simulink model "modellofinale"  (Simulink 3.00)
settings: Solver=ode45  StartTime=0.0  StopTime=10.0  RelTol=1e-3
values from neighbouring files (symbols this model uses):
  a = u(9)    [acceler.m]    (also in Dati2lin.m = 1; cin_inversa.m = u(4))
  b1 = 1    [Dati2lin.m]
  b2 = 1    [Dati2lin.m]
  Del1 = 0.0022    [Dati2lin.m]
  Del2 = 0.0022    [Dati2lin.m]
  Dm1 = 0.000172    [Dati2lin.m]
  Dm2 = 0.000071    (= 7.1e-05)    [Dati2lin.m]
  g = u(10)    [acceler.m]    (also in Dati2lin.m = 9.806)
  Jm1 = 0.000656    [Dati2lin.m]
  Jm2 = 0.000027    (= 2.7e-05)    [Dati2lin.m]
  Kcp1 = 32    [Dati2lin.m]
  Kcp2 = 32    [Dati2lin.m]
  Kcv1 = 0.24275    [Dati2lin.m]
  Kcv2 = 0.029363    [Dati2lin.m]
  Kel1 = 36.3    [Dati2lin.m]
  Kel2 = 4.6    [Dati2lin.m]
  Kt1 = 1.75    [Dati2lin.m]
  Kt2 = 0.97    [Dati2lin.m]
  m1 = u(7)    [acceler.m]    (also in Dati2lin.m = 19)
  m2 = u(8)    [acceler.m]    (also in Dati2lin.m = 9)
  n1 = 100    [Dati2lin.m]
  n2 = 100    [Dati2lin.m]
  q01 = atan2(s1,c1)    [traiettoria1.m]    (also in traiettoria2.m; traiettoria3.m; Dati2lin.m = 0)
  q02 = atan2(s2,c2)    [traiettoria1.m]    (also in traiettoria2.m; traiettoria3.m; Dati2lin.m = 0)
  qm01 = n1*q01 + taulm01/Kel1    [traiettoria1.m]    (also in traiettoria2.m; traiettoria3.m; Dati2lin.m)
  qm02 = n2*q02 + taulm02/Kel2    [traiettoria1.m]    (also in traiettoria2.m; traiettoria3.m; Dati2lin.m)
  Tiv1 = 25    [Dati2lin.m]
  Tiv2 = 5.2632    [Dati2lin.m]
  u01 = taulm01/Kt1    [traiettoria1.m]    (also in traiettoria2.m; traiettoria3.m; Dati2lin.m)
  u02 = taulm02/Kt2    [traiettoria1.m]    (also in traiettoria2.m; traiettoria3.m; Dati2lin.m)

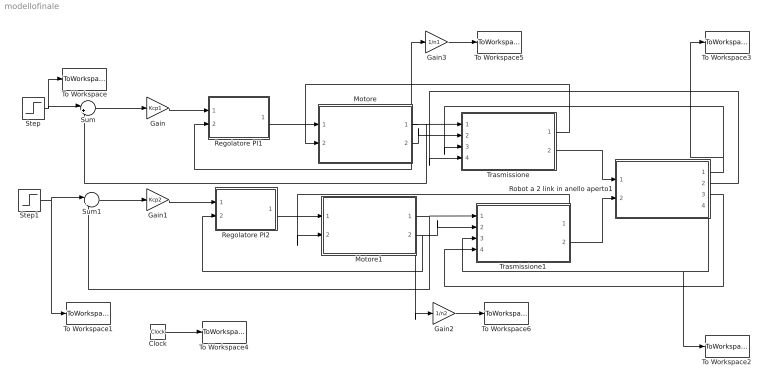
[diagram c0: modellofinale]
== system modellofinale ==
  Clock : Clock
  Gain : Gain  Gain=Kcp1  SaturateOnIntegerOverflow=on
  Gain1 : Gain  Gain=Kcp2  SaturateOnIntegerOverflow=on
  Gain2 : Gain  Gain=1/n2  SaturateOnIntegerOverflow=on
  Gain3 : Gain  Gain=1/n1  SaturateOnIntegerOverflow=on
  Motore : Subsystem  mask(Motore (solo meccanica)){Kt=Kt1, Jm=Jm1, Dm=Dm1, Qm0=qm01}
      mask prompts: Kt "Costante di coppia (Kt)"; Jm "Momento d'inerzia (Jm)"; Dm "Coefficiente di attrito viscoso (Dm)"; Qm0 "Posizione iniziale (Qm0)"
      mask help: Motore controllato in tensione - Modello che tiene conto degli effetti dell'attrito (solo quello viscoso)
  Motore1 : Subsystem  mask(Motore (solo meccanica)){Kt=Kt2, Jm=Jm2, Dm=Dm2, Qm0=qm02}
      mask prompts: Kt "Costante di coppia (Kt)"; Jm "Momento d'inerzia (Jm)"; Dm "Coefficiente di attrito viscoso (Dm)"; Qm0 "Posizione iniziale (Qm0)"
      mask help: Motore controllato in tensione - Modello che tiene conto degli effetti dell'attrito (solo quello viscoso)
  Regolatore PI1 : Subsystem  mask(Controllore PID ISA){Kc=Kcv1, Ti=Tiv1, b=b1, p6=[-inf,inf], u0=u01}
      mask prompts: Kc "Guadagno (Kc)"; Ti "Tempo integrale (Ti)"; b "Peso sul setpoint (b)"; p6 "Saturazione antiwindup ([umin, umax])"; u0 "Variabile di controllo iniziale (u0)"
      mask init:
      | ulow = p6(1);
      | uhigh = p6(2);
  Regolatore PI2 : Subsystem  mask(Controllore PID ISA){Kc=Kcv2, Ti=Tiv2, b=b2, p6=[-inf,inf], u0=u02}
      mask prompts: Kc "Guadagno (Kc)"; Ti "Tempo integrale (Ti)"; b "Peso sul setpoint (b)"; p6 "Saturazione antiwindup ([umin, umax])"; u0 "Variabile di controllo iniziale (u0)"
      mask init:
      | ulow = p6(1);
      | uhigh = p6(2);
  Robot a 2 link in anello aperto1 : Subsystem  mask(Modello del robot planare a 2 link){m1=m1, m2=m2, a=a, q01=q01, q02=q02, g=g}
      mask prompts: m1 "Massa del link 1 (m1)"; m2 "Massa del link 2 (m2)"; a "Lunghezza del link (a)"; q01 "Posizione iniziale link 1 (q01)"; q02 "Posizione iniziale link 2 (q02)"; g "Accelerazione di gravità (g)"
  Step : Step  Time=0  Before=0  After=0  SampleTime=0
  Step1 : Step  Time=0.1  Before=0  After=n2  SampleTime=0
  Sum : Sum  Inputs=|+-  SaturateOnIntegerOverflow=on
  Sum1 : Sum  Inputs=|+-  SaturateOnIntegerOverflow=on
  To Workspace : ToWorkspace  VariableName=step1  SampleTime=-1  SaveFormat=Matrix
  To Workspace1 : ToWorkspace  VariableName=step2  SampleTime=-1  SaveFormat=Matrix
  To Workspace2 : ToWorkspace  VariableName=qout2  SampleTime=-1  SaveFormat=Matrix
  To Workspace3 : ToWorkspace  VariableName=qout1  SampleTime=-1  SaveFormat=Matrix
  To Workspace4 : ToWorkspace  VariableName=x  SampleTime=-1  SaveFormat=Matrix
  To Workspace5 : ToWorkspace  VariableName=qmout1  SampleTime=-1  SaveFormat=Matrix
  To Workspace6 : ToWorkspace  VariableName=qmout2  SampleTime=-1  SaveFormat=Matrix
  Trasmissione : Subsystem  mask(Riduttore){n=n1, Kel=Kel1, Del=Del1}
      mask prompts: n "Rapporto di trasmissione (n)"; Kel "Coefficiente di elasticità (Kel)"; Del "Coefficiente di smorzamento (Del)"
      mask help: Riduttore - Modello che tiene conto dei soli effetti elastici (senza considerare le inerzie, accorpate nel modello del motore) e di un termine di smorzamento
  Trasmissione1 : Subsystem  mask(Riduttore){n=n2, Kel=Kel2, Del=Del2}
      mask prompts: n "Rapporto di trasmissione (n)"; Kel "Coefficiente di elasticità (Kel)"; Del "Coefficiente di smorzamento (Del)"
      mask help: Riduttore - Modello che tiene conto dei soli effetti elastici (senza considerare le inerzie, accorpate nel modello del motore) e di un termine di smorzamento
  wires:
  Sum/1 -> Gain/1
  Sum1/1 -> Gain1/1
  Gain/1 -> Regolatore PI1/1(ysp)
  Gain1/1 -> Regolatore PI2/1(ysp)
  Regolatore PI1/1(u) -> Motore/1(I)
  Regolatore PI2/1(u) -> Motore1/1(I)
  Trasmissione/2("tau_ll ") -> Robot a 2 link in anello aperto1/1(taull1)
  Trasmissione1/2("tau_ll ") -> Robot a 2 link in anello aperto1/2(taull2)
  Trasmissione1/1("tau_lm ") -> Motore1/2(tau_lm)
  Robot a 2 link in anello aperto1/3(dq2) -> Trasmissione1/4("dq ")
  Robot a 2 link in anello aperto1/2(dq1) -> Trasmissione/4("dq ")
  Trasmissione/1("tau_lm ") -> Motore/2(tau_lm)
  Motore1/2(dqm) -> Trasmissione1/2(dqm), Regolatore PI2/2(y)
  Motore/2(dqm) -> Trasmissione/2(dqm), Regolatore PI1/2(y)
  Motore/1(qm) -> Trasmissione/1(qm), Sum/2, Gain3/1
  Motore1/1(qm) -> Trasmissione1/1(qm), Sum1/2, Gain2/1
  Step/1 -> Sum/1, To Workspace/1
  Step1/1 -> Sum1/1, To Workspace1/1
  Robot a 2 link in anello aperto1/1(q1) -> Trasmissione/3("q "), To Workspace3/1
  Robot a 2 link in anello aperto1/4(q2) -> Trasmissione1/3("q "), To Workspace2/1
  Clock/1 -> To Workspace4/1
  Gain3/1 -> To Workspace5/1
  Gain2/1 -> To Workspace6/1

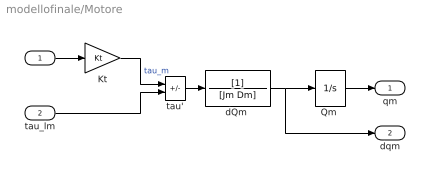
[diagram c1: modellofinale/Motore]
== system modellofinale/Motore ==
  I : Inport  Port=1  PortWidth=-1  SampleTime=-1  DataType=auto
  tau_lm : Inport  Port=2  PortWidth=-1  SampleTime=-1  DataType=auto
  Kt : Gain  Gain=Kt  SaturateOnIntegerOverflow=on
  "Qm " : Integrator  ExternalReset=none  InitialConditionSource=internal  InitialCondition=Qm0  LimitOutput=off  UpperSaturationLimit=inf  LowerSaturationLimit=-inf  ShowSaturationPort=off  ShowStatePort=off  AbsoluteTolerance=auto
  "dQm " : TransferFcn  Numerator=[1]  Denominator=[Jm Dm]
  tau' : Sum  Inputs=+-  SaturateOnIntegerOverflow=on
  qm : Outport  Port=1
  dqm : Outport  Port=2
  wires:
  "Qm "/1 -> qm/1
  "dQm "/1 -> dqm/1, "Qm "/1
  tau'/1 -> "dQm "/1
  Kt/1 -> tau'/1  "tau_m"
  I/1 -> Kt/1
  tau_lm/1 -> tau'/2

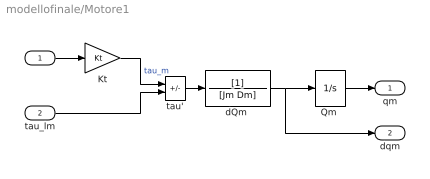
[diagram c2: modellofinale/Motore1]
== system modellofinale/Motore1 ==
  I : Inport  Port=1  PortWidth=-1  SampleTime=-1  DataType=auto
  tau_lm : Inport  Port=2  PortWidth=-1  SampleTime=-1  DataType=auto
  Kt : Gain  Gain=Kt  SaturateOnIntegerOverflow=on
  "Qm " : Integrator  ExternalReset=none  InitialConditionSource=internal  InitialCondition=Qm0  LimitOutput=off  UpperSaturationLimit=inf  LowerSaturationLimit=-inf  ShowSaturationPort=off  ShowStatePort=off  AbsoluteTolerance=auto
  "dQm " : TransferFcn  Numerator=[1]  Denominator=[Jm Dm]
  tau' : Sum  Inputs=+-  SaturateOnIntegerOverflow=on
  qm : Outport  Port=1
  dqm : Outport  Port=2
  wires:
  "Qm "/1 -> qm/1
  "dQm "/1 -> dqm/1, "Qm "/1
  tau'/1 -> "dQm "/1
  Kt/1 -> tau'/1  "tau_m"
  I/1 -> Kt/1
  tau_lm/1 -> tau'/2

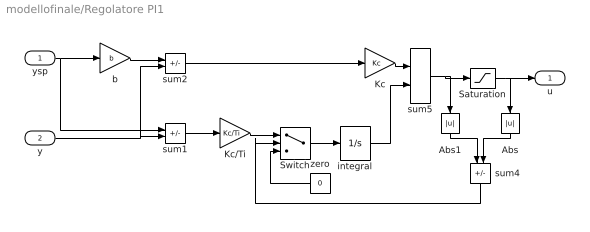
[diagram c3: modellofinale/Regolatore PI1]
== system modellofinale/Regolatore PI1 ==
  ysp : Inport  Port=1  PortWidth=-1  SampleTime=-1  DataType=auto
  y : Inport  Port=2  PortWidth=-1  SampleTime=-1  DataType=auto
  Abs : Abs  Orientation=down
  Abs1 : Abs  Orientation=down
  Kc : Gain  Gain=Kc  SaturateOnIntegerOverflow=on
  Kc/Ti : Gain  Gain=Kc/Ti  SaturateOnIntegerOverflow=on
  Saturation : Saturate  UpperLimit=uhigh  LowerLimit=ulow
  Switch : Switch  Threshold=0
  b : Gain  Gain=b  SaturateOnIntegerOverflow=on
  integral : Integrator  ExternalReset=none  InitialConditionSource=internal  InitialCondition=u0  LimitOutput=off  UpperSaturationLimit=inf  LowerSaturationLimit=-inf  ShowSaturationPort=off  ShowStatePort=off  AbsoluteTolerance=auto
  sum1 : Sum  Inputs=+-  SaturateOnIntegerOverflow=on
  sum2 : Sum  Inputs=+-  SaturateOnIntegerOverflow=on
  sum4 : Sum  Orientation=down  Inputs=-+  SaturateOnIntegerOverflow=on
  sum5 : Sum  Inputs=++  SaturateOnIntegerOverflow=on
  zero : Constant  Orientation=left  Value=0
  u : Outport  Port=1
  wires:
  integral/1 -> sum5/2
  sum1/1 -> Kc/Ti/1
  Abs/1 -> sum4/2
  Abs1/1 -> sum4/1
  sum5/1 -> Saturation/1, Abs1/1
  Saturation/1 -> Abs/1, u/1
  Switch/1 -> integral/1
  zero/1 -> Switch/3
  sum4/1 -> Switch/2
  Kc/Ti/1 -> Switch/1
  Kc/1 -> sum5/1
  sum2/1 -> Kc/1
  y/1 -> sum1/2, sum2/2
  b/1 -> sum2/1
  ysp/1 -> sum1/1, b/1

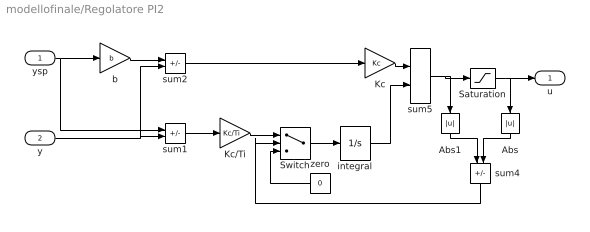
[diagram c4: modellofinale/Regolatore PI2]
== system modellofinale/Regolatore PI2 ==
  ysp : Inport  Port=1  PortWidth=-1  SampleTime=-1  DataType=auto
  y : Inport  Port=2  PortWidth=-1  SampleTime=-1  DataType=auto
  Abs : Abs  Orientation=down
  Abs1 : Abs  Orientation=down
  Kc : Gain  Gain=Kc  SaturateOnIntegerOverflow=on
  Kc/Ti : Gain  Gain=Kc/Ti  SaturateOnIntegerOverflow=on
  Saturation : Saturate  UpperLimit=uhigh  LowerLimit=ulow
  Switch : Switch  Threshold=0
  b : Gain  Gain=b  SaturateOnIntegerOverflow=on
  integral : Integrator  ExternalReset=none  InitialConditionSource=internal  InitialCondition=u0  LimitOutput=off  UpperSaturationLimit=inf  LowerSaturationLimit=-inf  ShowSaturationPort=off  ShowStatePort=off  AbsoluteTolerance=auto
  sum1 : Sum  Inputs=+-  SaturateOnIntegerOverflow=on
  sum2 : Sum  Inputs=+-  SaturateOnIntegerOverflow=on
  sum4 : Sum  Orientation=down  Inputs=-+  SaturateOnIntegerOverflow=on
  sum5 : Sum  Inputs=++  SaturateOnIntegerOverflow=on
  zero : Constant  Orientation=left  Value=0
  u : Outport  Port=1
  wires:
  integral/1 -> sum5/2
  sum1/1 -> Kc/Ti/1
  Abs/1 -> sum4/2
  Abs1/1 -> sum4/1
  sum5/1 -> Saturation/1, Abs1/1
  Saturation/1 -> Abs/1, u/1
  Switch/1 -> integral/1
  zero/1 -> Switch/3
  sum4/1 -> Switch/2
  Kc/Ti/1 -> Switch/1
  Kc/1 -> sum5/1
  sum2/1 -> Kc/1
  y/1 -> sum1/2, sum2/2
  b/1 -> sum2/1
  ysp/1 -> sum1/1, b/1

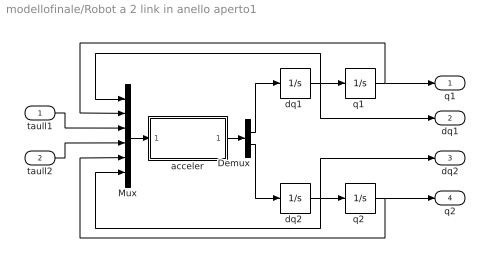
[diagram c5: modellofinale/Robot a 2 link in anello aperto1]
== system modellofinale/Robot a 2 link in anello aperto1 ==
  taull1 : Inport  Port=1  PortWidth=-1  SampleTime=-1  DataType=auto
  taull2 : Inport  Port=2  PortWidth=-1  SampleTime=-1  DataType=auto
  Demux : Demux  Outputs=2
  Mux : Mux  Inputs=6
  acceler : Subsystem
  "dq1 " : Integrator  ExternalReset=none  InitialConditionSource=internal  InitialCondition=0  LimitOutput=off  UpperSaturationLimit=inf  LowerSaturationLimit=-inf  ShowSaturationPort=off  ShowStatePort=off  AbsoluteTolerance=auto
  "dq2 " : Integrator  ExternalReset=none  InitialConditionSource=internal  InitialCondition=0  LimitOutput=off  UpperSaturationLimit=inf  LowerSaturationLimit=-inf  ShowSaturationPort=off  ShowStatePort=off  AbsoluteTolerance=auto
  "q1 " : Integrator  ExternalReset=none  InitialConditionSource=internal  InitialCondition=q01  LimitOutput=off  UpperSaturationLimit=inf  LowerSaturationLimit=-inf  ShowSaturationPort=off  ShowStatePort=off  AbsoluteTolerance=auto
  "q2 " : Integrator  ExternalReset=none  InitialConditionSource=internal  InitialCondition=q02  LimitOutput=off  UpperSaturationLimit=inf  LowerSaturationLimit=-inf  ShowSaturationPort=off  ShowStatePort=off  AbsoluteTolerance=auto
  q1 : Outport  Port=1
  dq1 : Outport  Port=2
  dq2 : Outport  Port=3
  q2 : Outport  Port=4
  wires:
  taull2/1 -> Mux/4
  taull1/1 -> Mux/3
  Mux/1 -> acceler/1(u)
  Demux/2 -> "dq2 "/1
  Demux/1 -> "dq1 "/1
  acceler/1(y) -> Demux/1
  "q2 "/1 -> Mux/5, q2/1
  "q1 "/1 -> Mux/2, q1/1
  "dq2 "/1 -> Mux/6, dq2/1, "q2 "/1
  "dq1 "/1 -> Mux/1, dq1/1, "q1 "/1

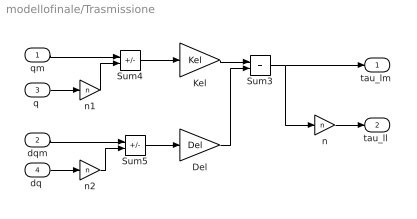
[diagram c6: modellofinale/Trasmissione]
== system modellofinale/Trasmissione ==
  qm : Inport  Port=1  PortWidth=-1  SampleTime=-1  DataType=auto
  dqm : Inport  Port=2  PortWidth=-1  SampleTime=-1  DataType=auto
  "q " : Inport  Port=3  PortWidth=-1  SampleTime=-1  DataType=auto
  "dq " : Inport  Port=4  PortWidth=-1  SampleTime=-1  DataType=auto
  Del : Gain  Gain=Del  SaturateOnIntegerOverflow=on
  Kel : Gain  Gain=Kel  SaturateOnIntegerOverflow=on
  Sum3 : Sum  Inputs=++  SaturateOnIntegerOverflow=on
  Sum4 : Sum  Inputs=+-  SaturateOnIntegerOverflow=on
  Sum5 : Sum  Inputs=+-  SaturateOnIntegerOverflow=on
  n : Gain  Gain=n  SaturateOnIntegerOverflow=on
  n1 : Gain  Gain=n  SaturateOnIntegerOverflow=on
  n2 : Gain  Gain=n  SaturateOnIntegerOverflow=on
  "tau_lm " : Outport  Port=1
  "tau_ll " : Outport  Port=2
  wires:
  Kel/1 -> Sum3/1
  Sum4/1 -> Kel/1
  n1/1 -> Sum4/2
  qm/1 -> Sum4/1
  Sum3/1 -> "tau_lm "/1, n/1
  Del/1 -> Sum3/2
  Sum5/1 -> Del/1
  n/1 -> "tau_ll "/1
  "q "/1 -> n1/1
  n2/1 -> Sum5/2
  dqm/1 -> Sum5/1
  "dq "/1 -> n2/1

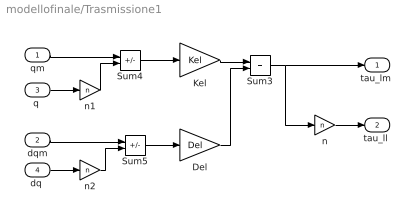
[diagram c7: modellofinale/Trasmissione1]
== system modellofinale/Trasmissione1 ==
  qm : Inport  Port=1  PortWidth=-1  SampleTime=-1  DataType=auto
  dqm : Inport  Port=2  PortWidth=-1  SampleTime=-1  DataType=auto
  "q " : Inport  Port=3  PortWidth=-1  SampleTime=-1  DataType=auto
  "dq " : Inport  Port=4  PortWidth=-1  SampleTime=-1  DataType=auto
  Del : Gain  Gain=Del  SaturateOnIntegerOverflow=on
  Kel : Gain  Gain=Kel  SaturateOnIntegerOverflow=on
  Sum3 : Sum  Inputs=++  SaturateOnIntegerOverflow=on
  Sum4 : Sum  Inputs=+-  SaturateOnIntegerOverflow=on
  Sum5 : Sum  Inputs=+-  SaturateOnIntegerOverflow=on
  n : Gain  Gain=n  SaturateOnIntegerOverflow=on
  n1 : Gain  Gain=n  SaturateOnIntegerOverflow=on
  n2 : Gain  Gain=n  SaturateOnIntegerOverflow=on
  "tau_lm " : Outport  Port=1
  "tau_ll " : Outport  Port=2
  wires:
  Kel/1 -> Sum3/1
  Sum4/1 -> Kel/1
  n1/1 -> Sum4/2
  qm/1 -> Sum4/1
  Sum3/1 -> "tau_lm "/1, n/1
  Del/1 -> Sum3/2
  Sum5/1 -> Del/1
  n/1 -> "tau_ll "/1
  "q "/1 -> n1/1
  n2/1 -> Sum5/2
  dqm/1 -> Sum5/1
  "dq "/1 -> n2/1

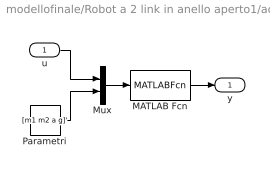
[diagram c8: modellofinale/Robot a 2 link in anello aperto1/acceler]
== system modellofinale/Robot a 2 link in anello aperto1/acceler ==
  u : Inport  Port=1  PortWidth=-1  SampleTime=-1  DataType=auto
  MATLAB Fcn : MATLABFcn  MATLABFcn=acceler  OutputWidth=-1  OutputSignalType=auto
  Mux : Mux  Inputs=2
  Parametri : Constant  Value=[m1 m2 a g]'
  y : Outport  Port=1
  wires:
  MATLAB Fcn/1 -> y/1
  Mux/1 -> MATLAB Fcn/1
  u/1 -> Mux/1
  Parametri/1 -> Mux/2
